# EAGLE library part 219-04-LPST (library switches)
SWITCH TAPE SEAL 4 POS SMD
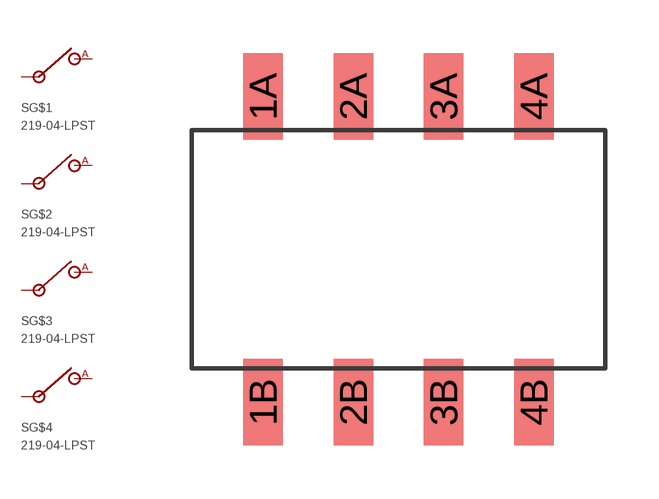
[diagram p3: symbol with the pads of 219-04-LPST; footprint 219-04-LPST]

Designator prefix S; gates G$1=SPST G$2=SPST G$3=SPST G$4=SPST

## 219-04-LPST (DIGIKEY: CT2194LPST-ND)  [219-04-LPST]
1A  G$1:A
1B  G$1:IN
2A  G$2:A
2B  G$2:IN
3A  G$3:A
3B  G$3:IN
4A  G$4:A
4B  G$4:IN

## Footprint 219-04-LPST (pad centres in mm)
4 switch dip switch bank, SPST
smd 1.118 x 2.438: 1A -3.81,4.305; 1B -3.81,-4.305; 2A -1.27,4.305; 2B -1.27,-4.305; 3A 1.27,4.305; 3B 1.27,-4.305; 4A 3.81,4.305; 4B 3.81,-4.305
